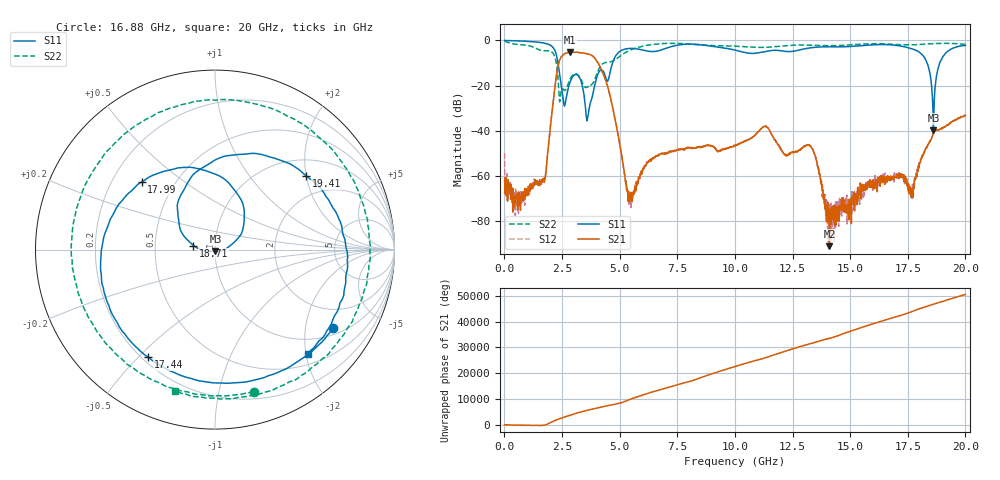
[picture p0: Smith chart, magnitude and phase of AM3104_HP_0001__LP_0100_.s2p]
!Created with skrf (http://scikit-rf.org).
# Hz S RI R 50.0
!freq ReS11 ImS11 ReS21 ImS21 ReS12 ImS12 ReS22 ImS22
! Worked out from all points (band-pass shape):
!   1601 points, 10 MHz to 20 GHz, reference 50 ohm
!   highest |S21| = -5.17 dB at 2.846 GHz (marker M1); lowest = -90.9 dB at 14.1 GHz (marker M2)
!   |S21| within 3 dB of the highest: 2.418 GHz to 3.949 GHz (1.531 GHz wide, 48.1 % of centre)
!   lowest |S11| = -39.8 dB at 18.61 GHz (marker M3), VSWR 1.02, Z = 50.3 - j0.997 ohm
!   |S11| at or under -10 dB: 2.326 GHz to 4.69 GHz (2.364 GHz wide, 67.4 % of centre); 18.34 GHz to 18.88 GHz (544.3 MHz wide, 2.92 % of centre)
!   |S22| runs from -27.1 to -0.2 dB; largest |S21 - S12| = 0.0037
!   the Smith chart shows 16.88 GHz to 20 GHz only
!   S11 on the Smith chart (normalised r, x): 16.88 GHz: 1.21, -2.83; 17.44 GHz: 0.22, -0.53; 17.99 GHz: 0.33, +0.36; 18.71 GHz: 0.79, +0.04; 19.41 GHz: 1.40, +2.00; 20 GHz: 0.69, -2.03
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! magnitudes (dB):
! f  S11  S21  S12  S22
! 10 MHz  0.0  -60.6  -49.7  -0.2
! 572.2 MHz  -0.2  -74.8  -67.5  -1.7
! 1.672 GHz  -1.0  -61.4  -61.2  -4.5
! 2.334 GHz  -10.5  -10.9  -10.9  -17.8
! 2.596 GHz  -28.8  -6.0  -6.0  -22.2
! 2.846 GHz  -18.5  -5.2  -5.2  -17.2
! 3.346 GHz  -18.6  -5.5  -5.5  -17.8
! 3.608 GHz  -34.2  -6.0  -6.0  -20.4
! 4.408 GHz  -16.7  -18.0  -18.0  -9.7
! 5.445 GHz  -3.5  -70.5  -69.7  -4.3
! 6.682 GHz  -4.5  -50.4  -50.4  -1.5
! 10.01 GHz  -4.2  -46.6  -46.2  -2.5
! 13.34 GHz  -3.1  -47.8  -47.4  -2.1
! 14.1 GHz  -2.8  -90.9  -72.9  -2.3
! 16.68 GHz  -1.9  -60.8  -61.6  -1.6
! 16.88 GHz  -2.0  -60.6  -61.5  -1.7
! 17.44 GHz  -3.0  -62.0  -62.3  -2.0
! 17.99 GHz  -5.1  -55.1  -54.9  -1.8
! 18.61 GHz  -39.8  -41.2  -41.1  -1.4
! 18.71 GHz  -18.3  -39.7  -40.0  -1.4
! 19.41 GHz  -3.7  -36.0  -35.9  -1.3
! 20 GHz  -2.2  -33.1  -33.1  -1.7
